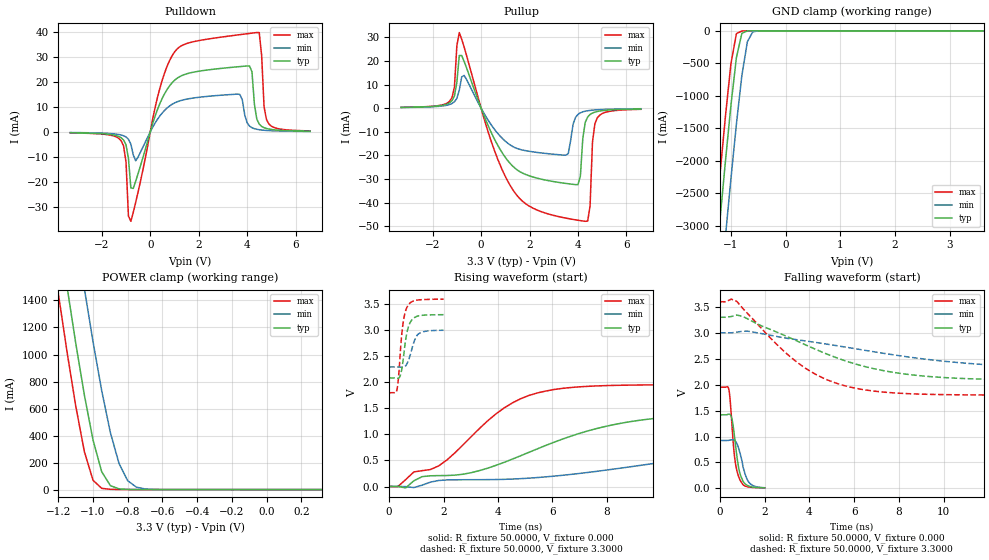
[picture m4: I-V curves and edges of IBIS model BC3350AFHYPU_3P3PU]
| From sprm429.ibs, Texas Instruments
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|   Model BC3350AFHYPU_3P3PU
[Model]   BC3350AFHYPU_3P3PU
Model_type   I/O
Polarity   Non-Inverting
Enable   Active-Low
Vinl =   0.9900V
Vinh =   2.3100V
Vmeas =   1.6500V
Cref =  15.0000pF
Rref = 100.0000M
Vref =  0.000V
C_comp   2.5478pF   2.6979pF   2.5389pF
[Temperature Range]   25.0000   0.1250k   -40.0000
[Voltage Range]   3.3000V   3.0000V   3.6000V
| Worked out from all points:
|   slope of the pulldown table from 0 to 0.495 V, typ, clamps not added: 36.7 ohm
|   slope of the pullup table from 0 to 0.495 V, typ, clamps not added: 41.5 ohm
|   GND clamp passes 1 mA (typ) near -0.67 V on its own axis
|   POWER clamp passes 1 mA (typ) near -0.78 V on its own axis
|   rising waveform, R_fixture 50.0000, V_fixture 0.000: 20-80 % time 4.65ns typ, 8.78ns min, 2.59ns max; typ from 0.002 V to 1.42 V
|   rising waveform, R_fixture 50.0000, V_fixture 3.3000: 20-80 % time 217ps typ, 266ps min, 190ps max; typ from 2.08 V to 3.29 V
|   falling waveform, R_fixture 50.0000, V_fixture 0.000: 20-80 % time 281ps typ, 337ps min, 247ps max; typ from 1.42 V to 0.011 V
|   falling waveform, R_fixture 50.0000, V_fixture 3.3000: 20-80 % time 4.41ns typ, 6.87ns min, 2.94ns max; typ from 3.3 V to 2.08 V
[Pulldown]
| voltage   I(typ)   I(min)   I(max)
-3.3V     -324uA     -232uA     -378uA
-1.2V     -2.324mA   -1.222mA   -3.542mA
-800mV    -22.44mA   -4.89mA    -35.82mA
-600mV    -19.72mA   -11.54mA   -28.19mA
300mV     9.042mA    5.104mA    13.91mA
1V        20.68mA    11.62mA    32.03mA
3.7V      26.21mA    15.05mA    39.01mA
4.1V      26.48mA    2.354mA    39.51mA
4.4V      5.156mA    1.069mA    39.85mA
4.5V      3.148mA    898.8uA    39.84mA
4.8V      1.388mA    604.9uA    4.95mA
6.6V      305uA      201uA      423uA
[Pullup]
| voltage   I(typ)   I(min)   I(max)
-3.3V     322uA      278uA      341uA
-1.3V     2.265mA    1.536mA    2.891mA
-900mV    22.26mA    7.57mA     31.99mA
600mV     -14.05mA   -9.585mA   -19.25mA
1.7V      -27.44mA   -17.71mA   -39.29mA
3.5V      -31.86mA   -19.91mA   -46.55mA
4V        -32.37mA   -2.653mA   -47.45mA
4.3V      -6.064mA   -1.298mA   -47.9mA
4.5V      -2.676mA   -959.1uA   -41.48mA
4.6V      -2.066mA   -847.2uA   -14.32mA
4.8V      -1.41mA    -686uA     -4.099mA
6.6V      -357uA     -250uA     -488uA
[GND_clamp]
| voltage   I(typ)   I(min)   I(max)
-3.3V     -23.37A    -24.46A    -22.74A
-1.3V     -3.836A    -5.005A    -3.135A
-1.2V     -2.907A    -4.076A    -2.207A
-1.1V     -2.003A    -3.163A    -1.312A
-1V       -1.147A    -2.276A    -506.5mA
-900mV    -411.7mA   -1.434A    -43.08mA
-800mV    -37.74mA   -687mA     -2.738mA
-700mV    -1.311mA   -169.2mA   -450.8uA
-600mV    -182.2uA   -14.71mA   -224.5uA
-400mV    -135.4uA   -133.8uA   -210.3uA
3.62V     0A         0A         0A
[POWER_clamp]
| voltage   I(typ)   I(min)   I(max)
-3.3V     22.31A     23.05A     21.9A
-1.2V     1.938A     2.775A     1.451A
-1.15V    1.504A     2.334A     1.021A
-1.1V     1.087A     1.904A     621.5mA
-1.05V    700.4mA    1.489A     281.6mA
-1V       367mA      1.095A     69.13mA
-950mV    132mA      732.5mA    9.408mA
-900mV    29.22mA    422.1mA    2.069mA
-850mV    5.457mA    192.5mA    1.019mA
-800mV    1.399mA    65.58mA    615.3uA
-650mV    171.2uA    1.376mA    146.1uA
320mV     0A         0A         0A
[Ramp]
| variable   typ   min   max
dV/dt_r   0.7919/4.1682n   0.2810/7.1658n   1.1673/2.5400n
dV/dt_f   0.6981/4.0247n   0.3310/4.8901n   1.0747/2.8761n
R_load = 50.0000
[Rising Waveform]
R_fixture = 50.0000
V_fixture = 0.000
V_fixture_min = 0.000
V_fixture_max = 0.000
| time   V(typ)   V(min)   V(max)
0s        2.434mV    2.071mV    2.815mV
606.1ps   -25.18mV   -1.573mV   132.6mV
1.212ns   189.7mV    26.12mV    304.7mV
1.818ns   209.6mV    116mV      395.1mV
4.546ns   529.5mV    144mV      1.608V
6.364ns   908mV      215.2mV    1.881V
8.788ns   1.237V     372.9mV    1.944V
11.82ns   1.378V     589.7mV    1.951V
18.18ns   1.417V     853mV      1.951V
30ns      1.419V     921.3mV    1.951V
[Rising Waveform]
R_fixture = 50.0000
V_fixture = 3.3000
V_fixture_min = 3.0000
V_fixture_max = 3.6000
| time   V(typ)   V(min)   V(max)
0s        2.082V     2.292V     1.798V
282.8ps   2.078V     2.293V     1.848V
343.4ps   2.078V     2.292V     2.09V
404ps     2.121V     2.289V     2.526V
505.1ps   2.392V     2.286V     3.107V
606.1ps   2.81V      2.315V     3.369V
686.9ps   3.022V     2.389V     3.467V
828.3ps   3.19V      2.624V     3.54V
1.051ns   3.268V     2.912V     3.575V
2ns       3.294V     2.995V     3.592V
[Falling Waveform]
R_fixture = 50.0000
V_fixture = 0.000
V_fixture_min = 0.000
V_fixture_max = 0.000
| time   V(typ)   V(min)   V(max)
0s        1.419V     924.4mV    1.951V
404ps     1.433V     928mV      1.893V
464.6ps   1.42V      933mV      1.65V
525.3ps   1.355V     937.3mV    1.286V
646.5ps   1.01V      926.3mV    628.8mV
747.5ps   647.8mV    871.6mV    357.9mV
868.7ps   329mV      722.1mV    189mV
1.03ns    135.2mV    415.5mV    71.46mV
1.273ns   48.02mV    130.1mV    27.86mV
2ns       11.32mV    13.05mV    10.58mV
[Falling Waveform]
R_fixture = 50.0000
V_fixture = 3.3000
V_fixture_min = 3.0000
V_fixture_max = 3.6000
| time   V(typ)   V(min)   V(max)
0s        3.3V       3V         3.6V
505.1ps   3.314V     2.999V     3.65V
757.6ps   3.343V     3.013V     3.604V
2.778ns   2.97V      2.91V      2.678V
4.04ns    2.727V     2.83V      2.258V
5.051ns   2.545V     2.764V     2.051V
6.313ns   2.368V     2.675V     1.911V
8.838ns   2.178V     2.51V      1.82V
12.63ns   2.096V     2.362V     1.8V
25ns      2.082V     2.293V     1.798V
